FUNCTION_BLOCK Example21_startupPMS //any amount of xbots 
VAR_INPUT
	Execute : BOOL;
END_VAR
VAR_OUTPUT
	Done : BOOL;
END_VAR
VAR_IN_OUT
	PM_Controller : PMControllerType;	// the planar motor controller to use
END_VAR
VAR
	PMC_StartUpPlanarMotorSystem1 : PMC_StartUpPlanarMotorSystem;
	xbotIDs : ARRAY[0..99] OF USINT;
	numXbots : USINT;
END_VAR

//any amount of xbots 

PMC_StartUpPlanarMotorSystem1(Execute := Execute,NumXbots => numXbots,Xbot_IDs => xbotIDs,PM_Controller := PM_Controller);

Done := PMC_StartUpPlanarMotorSystem1.Done;

END_FUNCTION_BLOCK
